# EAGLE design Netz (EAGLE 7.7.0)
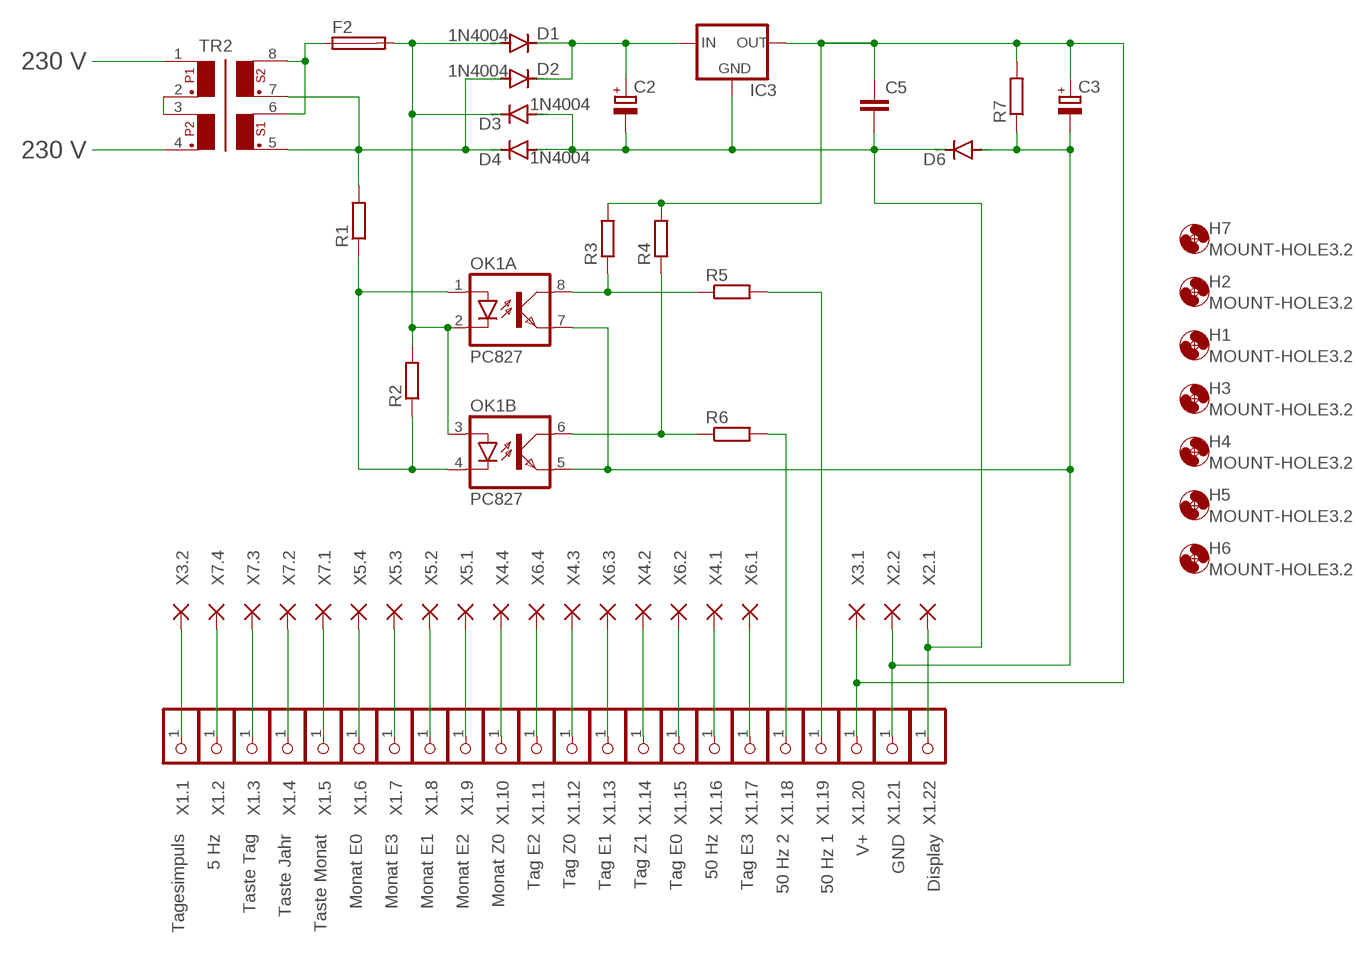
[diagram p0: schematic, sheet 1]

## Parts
C2  CPOL-EUE7.5-18  [E7,5-18]
C3  CPOL-EUE5-13  [E5-13]
C5  C-EU050-024X044  [C050-024X044]
D1  1N4004  [DO41-10]
D2  1N4004  [DO41-10]
D3  1N4004  [DO41-10]
D4  1N4004  [DO41-10]
D6  1N4148DO35-10  [DO35-10]
F2  SH22,5  [SH22,5]
H1  MOUNT-HOLE3.2  [3,2]
H2  MOUNT-HOLE3.2  [3,2]
H3  MOUNT-HOLE3.2  [3,2]
H4  MOUNT-HOLE3.2  [3,2]
H5  MOUNT-HOLE3.2  [3,2]
H6  MOUNT-HOLE3.2  [3,2]
H7  MOUNT-HOLE3.2  [3,2]
IC3  78XXS  [78XXS]
OK1  PC827  [DIL08]
R1  R-EU_0207/10  [0207/10]
R2  R-EU_0207/10  [0207/10]
R3  R-EU_0207/10  [0207/10]
R4  R-EU_0207/10  [0207/10]
R5  R-EU_0207/10  [0207/10]
R6  R-EU_0207/10  [0207/10]
R7  R-EU_0207/10  [0207/10]
TR2  FL02  [FL02-08]
X1.1  Tagesimpuls  PINHD-1X1  [1X01]
X1.2  5 Hz  PINHD-1X1  [1X01]
X1.3  Taste Tag  PINHD-1X1  [1X01]
X1.4  Taste Jahr  PINHD-1X1  [1X01]
X1.5  Taste Monat  PINHD-1X1  [1X01]
X1.6  Monat E0  PINHD-1X1  [1X01]
X1.7  Monat E3  PINHD-1X1  [1X01]
X1.8  Monat E1  PINHD-1X1  [1X01]
X1.9  Monat E2  PINHD-1X1  [1X01]
X1.10  Monat Z0  PINHD-1X1  [1X01]
X1.11  Tag E2  PINHD-1X1  [1X01]
X1.12  Tag Z0  PINHD-1X1  [1X01]
X1.13  Tag E1  PINHD-1X1  [1X01]
X1.14  Tag Z1  PINHD-1X1  [1X01]
X1.15  Tag E0  PINHD-1X1  [1X01]
X1.16  50 Hz  PINHD-1X1  [1X01]
X1.17  Tag E3  PINHD-1X1  [1X01]
X1.18  50 Hz 2  PINHD-1X1  [1X01]
X1.19  50 Hz 1  PINHD-1X1  [1X01]
X1.20  V+  PINHD-1X1  [1X01]
X1.21  GND  PINHD-1X1  [1X01]
X1.22  Display  PINHD-1X1  [1X01]
X2.1  WIREPAD1,6/0,8  [1,6/0,8]
X2.2  WIREPAD1,6/0,8  [1,6/0,8]
X3.1  WIREPAD1,6/0,8  [1,6/0,8]
X3.2  WIREPAD1,6/0,8  [1,6/0,8]
X4.1  WIREPAD1,6/0,8  [1,6/0,8]
X4.2  WIREPAD1,6/0,8  [1,6/0,8]
X4.3  WIREPAD1,6/0,8  [1,6/0,8]
X4.4  WIREPAD1,6/0,8  [1,6/0,8]
X5.1  WIREPAD1,6/0,8  [1,6/0,8]
X5.2  WIREPAD1,6/0,8  [1,6/0,8]
X5.3  WIREPAD1,6/0,8  [1,6/0,8]
X5.4  WIREPAD1,6/0,8  [1,6/0,8]
X6.1  WIREPAD1,6/0,8  [1,6/0,8]
X6.2  WIREPAD1,6/0,8  [1,6/0,8]
X6.3  WIREPAD1,6/0,8  [1,6/0,8]
X6.4  WIREPAD1,6/0,8  [1,6/0,8]
X7.1  WIREPAD1,6/0,8  [1,6/0,8]
X7.2  WIREPAD1,6/0,8  [1,6/0,8]
X7.3  WIREPAD1,6/0,8  [1,6/0,8]
X7.4  WIREPAD1,6/0,8  [1,6/0,8]

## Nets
N$1: D1.A D3.C F2.2 OK1.2(A:C) OK1.3(B:A) R2.2
N$2: F2.1 TR2.6 TR2.8
N$3: R5.2 X1.19.1
N$4: D2.A D4.C R1.2 TR2.5 TR2.7
N$5: C2.+ D1.C D2.C IC3.IN
N$6: R6.2 X1.18.1
N$7: X1.11.1 X6.4.1(P)
N$9: TR2.2 TR2.3
N$10: TR2.1
N$11: TR2.4
N$12: OK1.1(A:A) OK1.4(B:C) R1.1 R2.1
N$13: X1.13.1 X6.3.1(P)
N$14: OK1.8(A:COL) R3.1 R5.1
N$15: C2.- C5.2 D3.A D4.A D6.C IC3.GND X1.22.1 X2.1.1(P)
N$16: OK1.6(B:COL) R4.1 R6.1
N$17: C3.+ C5.1 IC3.OUT R3.2 R4.2 R7.2 X1.20.1 X3.1.1(P)
N$18: X1.15.1 X6.2.1(P)
N$19: X1.14.1 X4.2.1(P)
N$20: X1.12.1 X4.3.1(P)
N$21: X1.17.1 X6.1.1(P)
N$22: X1.16.1 X4.1.1(P)
N$23: X1.10.1 X4.4.1(P)
N$24: X1.6.1 X5.4.1(P)
N$25: X1.7.1 X5.3.1(P)
N$26: X1.8.1 X5.2.1(P)
N$27: X1.9.1 X5.1.1(P)
N$28: X1.4.1 X7.2.1(P)
N$29: X1.1.1 X3.2.1(P)
N$30: X1.5.1 X7.1.1(P)
N$31: X1.3.1 X7.3.1(P)
N$32: X1.2.1 X7.4.1(P)
N$33: C3.- D6.A OK1.5(B:EMIT) OK1.7(A:EMIT) R7.1 X1.21.1 X2.2.1(P)

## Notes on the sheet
- 230 V
- 230 V

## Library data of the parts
C2 C3 = rclxrund:CPOL-EU: POLARIZED CAPACITOR, European symbol; SPICEPREFIX: C
C5 = rclxrund:C-EU: CAPACITOR, European symbol; SPICEPREFIX: C
D1-D4 = diodexrund:1N4004: DIODE
D6 = diodexrund:1N4148: DIODE
F2 = fuserund:SH22,5: FUSE HOLDER; MF: SCHURTER; MPN: 0031.8201; OC_FARNELL: 1162740; OC_NEWARK: 96F8317
H1-H7 = holes:MOUNT-HOLE: MOUNTING HOLE with drill center marker
IC3 = v-regrund:78XXS: VOLTAGE REGULATOR
OK1 = optocouplerxrund:PC827: SHARP OPTO COUPLER; OC_FARNELL: unknown; OC_NEWARK: unknown
R1-R7 = rclxrund:R-EU_: RESISTOR, European symbol; SPICEPREFIX: R
TR2 = trafox:FL02: TRANSFORMER 2 primary winding, 2 secondary windings, mounting holes BLOCK
X1.1-X1.22 = pinheadxrund:PINHD-1X1: PIN HEADER
X2.1 X2.2 X3.1 X3.2 X4.1-X4.4 X5.1-X5.4 X6.1-X6.4 X7.1-X7.4 = wirepad:WIREPAD: Wire PAD connect wire on PCB

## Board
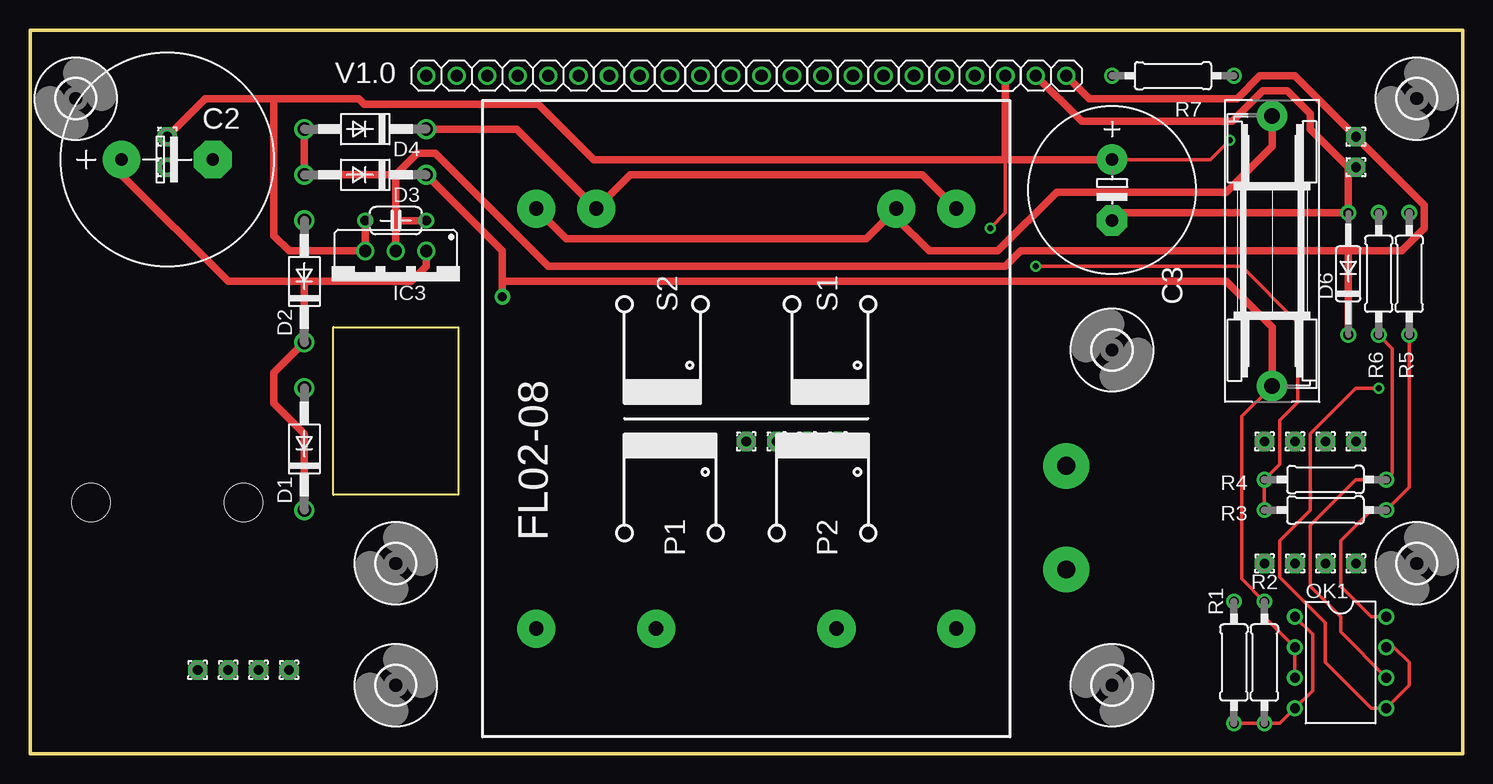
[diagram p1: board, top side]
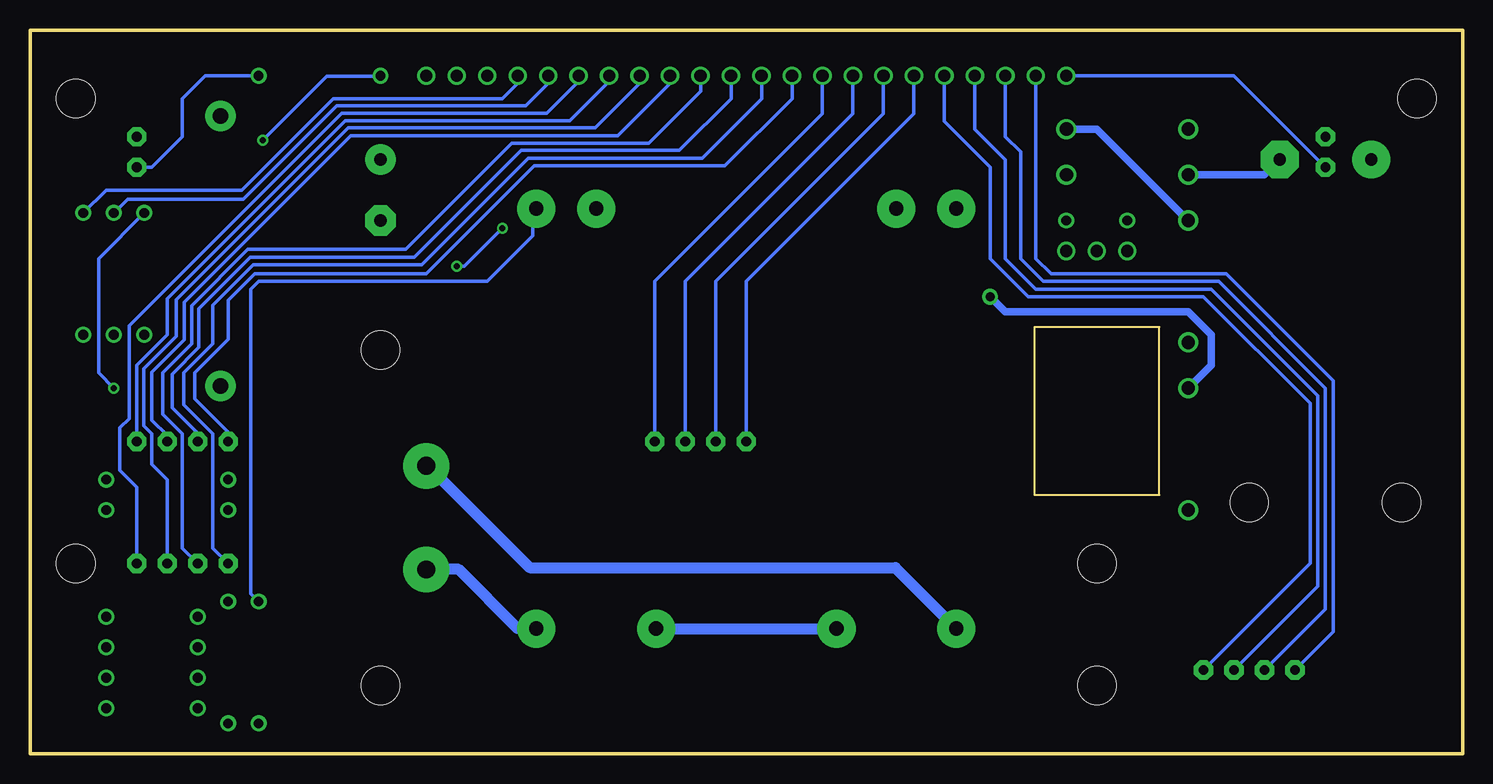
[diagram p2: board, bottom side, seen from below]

Size 119.38 x 60.33 mm. Coordinates in mm from the lower left corner, seen from the top.
Outline: 0,0 119.38,0 119.38,60.33 0,60.33 0,0
Copper layers (1*16): Top 0.035mm / dielectric 1.5mm / Bottom 0.035mm
Design rules "12mil": minimum track width 12mil, minimum drill 0.5mm, track to track 12mil, track to pad 12mil, pad to pad 12mil, via to via 12mil, smd to smd 6mil, copper to edge 40mil, drill to drill 12mil, minimum pad ring 10mil, minimum via ring 8mil, stop-mask expansion 4mil, vias tented up to drill 0mil, thermal gap 10mil
Holes 3.17 mm at 5.08,20.95 17.78,20.95
Milling: 4 lines

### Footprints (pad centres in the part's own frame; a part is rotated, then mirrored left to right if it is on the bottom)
E7,5-18 = drill 1.016 pad 3.15: + -3.81,0 | drill 1.016 pad 3.15 octagon: - 3.81,0
E5-13 = drill 1.016 pad 2.54: + -2.54,0 | drill 1.016 pad 2.54 octagon: - 2.54,0
C050-024X044 = drill 0.813: 1 -2.54,0; 2 2.54,0
DO41-10 = drill 1.118: A 5.08,0; C -5.08,0
DO35-10 = drill 0.813: A 5.08,0; C -5.08,0
SH22,5 = drill 1.321 pad 2.54: 1 -11.252,0; 2 11.252,0
3,2 = hole 3.2: 0,0
78XXS = drill 1.016: GND 0,-2.54; IN -2.54,-2.54; OUT 2.54,-2.54
DIL08 = drill 0.813: 1 -3.81,-3.81; 2 -1.27,-3.81; 3 1.27,-3.81; 4 3.81,-3.81; 5 3.81,3.81; 6 1.27,3.81; 7 -1.27,3.81; 8 -3.81,3.81
0207/10 = drill 0.813: 1 -5.08,0; 2 5.08,0
FL02-08 = drill 1.194 pad 3.175: 1 -17.501,17.501; 2 -17.501,7.518; 3 -17.501,-7.518; 4 -17.501,-17.501; 5 17.501,-17.501; 6 17.501,-12.497; 7 17.501,12.497; 8 17.501,17.501
1X01 = drill 1.016: 1 0,0
1,6/0,8 = drill 0.813 pad 1.6 octagon: 1 0,0

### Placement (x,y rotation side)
C2  11.43,49.53 0 top
C3  90.17,46.99 270 top
C5  30.48,44.45 0 top
D1  22.86,25.4 90 top
D2  22.86,39.37 90 top
D3  27.94,48.26 180 top
D4  27.94,52.07 180 top
D6  109.86,40.01 90 top
F2  103.5,41.91 270 top
H1  30.48,15.88 0 top
H2  30.48,5.71 0 top
H3  3.81,54.61 0 top
H4  115.57,54.61 0 top
H5  90.17,5.71 90 top
H6  90.17,33.66 90 top
H7  115.57,15.88 0 top
IC3  30.48,39.37 180 top
OK1  109.22,7.62 270 top
R1  100.33,7.62 90 top
R2  102.87,7.62 90 top
R3  107.95,20.32 180 top
R4  107.95,22.86 180 top
R5  114.94,40.01 90 top
R6  112.39,40.01 90 top
R7  95.25,56.52 180 top
TR2  59.69,27.94 90 top
X1.1  33.02,56.52 0 top
X1.2  35.56,56.52 0 top
X1.3  38.1,56.52 0 top
X1.4  40.64,56.52 0 top
X1.5  43.18,56.52 0 top
X1.6  45.72,56.52 0 top
X1.7  48.26,56.52 90 top
X1.8  50.8,56.52 90 top
X1.9  53.34,56.52 90 top
X1.10  55.88,56.52 90 top
X1.11  58.42,56.52 90 top
X1.12  60.96,56.52 90 top
X1.13  63.5,56.52 90 top
X1.14  66.04,56.52 90 top
X1.15  68.58,56.52 90 top
X1.16  71.12,56.52 90 top
X1.17  73.66,56.52 90 top
X1.18  76.2,56.52 180 top
X1.19  78.74,56.52 180 top
X1.20  81.28,56.52 90 top
X1.21  83.82,56.52 180 top
X1.22  86.36,56.52 90 top
X2.1  110.49,51.44 0 top
X2.2  110.49,48.9 0 top
X3.1  11.43,51.44 0 top
X3.2  11.43,48.9 0 top
X4.1  110.49,26.04 0 top
X4.2  107.95,26.04 0 top
X4.3  105.41,26.04 0 top
X4.4  102.87,26.04 0 top
X5.1  67.31,26.04 0 top
X5.2  64.77,26.04 0 top
X5.3  62.23,26.04 0 top
X5.4  59.69,26.04 0 top
X6.1  110.49,15.88 0 top
X6.2  107.95,15.88 0 top
X6.3  105.41,15.88 0 top
X6.4  102.87,15.88 0 top
X7.1  21.59,6.99 0 top
X7.2  19.05,6.99 0 top
X7.3  16.51,6.99 0 top
X7.4  13.97,6.99 0 top

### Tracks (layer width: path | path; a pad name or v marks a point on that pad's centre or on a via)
N$1  (via drill 0.75 pad 1.3)
  Top 0.305: F2.2 100.97,28.12 100.97,14.61 R2.2 102.87,11.43 OK1.2 OK1.3
  Top 0.61: D3.C 39.37,41.91 39.37,39.37 | v39.37,38.1 39.37,39.37 | F2.2 103.5,35.56 99.69,39.37 39.37,39.37
  Bottom 0.61: v39.37,38.1 38.1,36.83 22.86,36.83 20.95,34.92 20.95,32.38 D1.A
N$2
  Top 0.61: TR2.8 44.69,42.94 69.69,42.94 TR2.6 72.19,44.65 74.93,41.91 80.64,41.91 85.55,46.81 99.69,46.81 103.5,50.62 F2.1
N$3
  Bottom 0.305: X1.19.1 78.74,55.88 80.01,54.61 94.11,54.61 101.73,46.99 113.03,46.99 R5.2
N$4
  Top 0.61: TR2.5 74.37,48.26 50.01,48.26 TR2.7 40.56,52.07 D4.C
  Bottom 0.305: R1.2 100.97,13.34 100.97,38.73 100.33,39.37 81.28,39.37 77.47,43.18 77.47,45.16 TR2.5
  Bottom 0.61: D2.A 30.48,52.07 D4.C
N$5
  Top 0.61: IC3.IN 33.02,40.64 31.75,39.37 22.86,39.37 | 22.86,39.37 D2.C 20.32,31.75 20.32,29.21 22.86,26.67 D1.C | 22.86,39.37 16.51,39.37 7.62,48.26 C2.+
N$6
  Bottom 0.305: R6.2 112.37,45.09 111.23,46.23 101.6,46.23 93.83,54 78.08,54 76.2,55.88 X1.18.1
N$7
  Bottom 0.305: X6.4.1 104.14,17.14 104.14,26.7 106.55,29.11 106.55,31.75 104.14,34.16 104.14,37.39 100.77,40.77 86.74,40.77 77.85,49.66 63.37,49.66 58.42,54.61 X1.11.1
N$9
  Bottom 0.914: TR2.3 TR2.2
N$10  (via drill 1.5 pad 3.81)
  Bottom 0.914: TR2.1 47.27,15.52 77.75,15.52 86.23,24 v86.36,24
N$11  (via drill 1.5 pad 3.81)
  Bottom 0.914: TR2.4 78.74,10.44 83.67,15.37 v86.36,15.37
N$12
  Top 0.305: OK1.1 106.88,9.96 106.88,5.28 OK1.4 104.14,2.54 R2.1 R1.1
N$13
  Bottom 0.305: X1.13.1 63.5,55.22 67.82,50.9 79.22,50.9 88.08,42.04 101.22,42.04 105.92,37.34 105.92,34.16 108.33,31.75 108.33,28.32 106.68,26.67 106.68,17.14 X6.3.1
N$14
  Top 0.305: R5.1 114.94,22.23 R3.1 111.76,20.32 109.22,17.78 109.22,13.97 111.76,11.43 OK1.8
N$15
  Top 0.61: IC3.GND 30.48,44.45 | D4.A D3.A 30.48,48.26 | 30.48,44.45 C5.2 | 30.48,44.45 30.48,48.26 | 109.86,41.91 D6.C | 109.86,41.91 82.55,41.91 81.28,40.64 43.18,40.64 33.78,50.04 32.26,50.04 30.48,48.26 | 109.86,41.91 114.3,41.91 116.2,43.81 116.2,45.72 X2.1.1 105.41,56.52 102.49,56.52 100.58,54.61 88.27,54.61 X1.22.1
  Bottom 0.61: D3.A 16.51,48.26 C2.-
N$16
  Top 0.305: R6.1 113.54,33.78 113.54,23.37 R4.1 110.49,22.86 106.68,19.05 106.68,13.97 109.22,11.43 109.22,10.16 OK1.6
N$17  (via drill 0.5)
  Top 0.305: R3.2 R4.2 104.14,24.13 104.14,27.78 105.66,29.31 105.66,35.94 100.97,40.64 v83.82,40.64 | 81.28,49.53 81.28,45.09 v80.01,43.81 | v99.98,51.15 98.37,49.53 C3.+
  Top 0.61: C5.1 IC3.OUT 21.59,41.91 20.32,43.18 20.32,54.61 | C3.+ 81.28,49.53 | 81.28,49.53 46.99,49.53 42.37,54.15 27.86,54.15 27.4,54.61 20.32,54.61 | X1.20.1 81.28,49.53 | 20.32,54.61 14.61,54.61 X3.1.1
  Bottom 0.305: v83.82,40.64 83.19,40.64 v80.01,43.81 | v99.98,51.15 94.65,56.48 90.21,56.48 R7.2
N$18
  Bottom 0.305: X1.15.1 68.58,55.88 72.29,52.17 92.86,52.17 107.19,37.85 107.19,34.8 109.88,32.11 109.88,27.33 109.22,26.67 109.22,24.13 107.95,22.86 X6.2.1
N$19
  Bottom 0.305: X1.14.1 66.04,55.88 70.41,51.51 92.66,51.51 106.53,37.65 106.53,34.52 109.22,31.82 109.22,27.81 107.95,26.54 X4.2.1
N$20
  Bottom 0.305: X4.3.1 105.41,26.72 107.54,28.86 107.54,31.65 105.31,33.88 105.31,37.09 101.02,41.38 87.38,41.38 78.46,50.29 65.28,50.29 60.96,54.61 X1.12.1
N$21
  Bottom 0.305: X6.1.1 110.49,22.23 111.89,23.62 111.89,27.18 111.12,27.94 111.12,35.69 93.42,53.39 76.33,53.39 73.66,56.06 X1.17.1
N$22
  Bottom 0.305: X4.1.1 110.49,32.38 107.95,34.92 107.95,37.95 93.12,52.78 74.4,52.78 71.12,56.06 X1.16.1
N$23
  Bottom 0.305: X4.4.1 102.87,26.8 105.66,29.59 105.66,31.75 102.87,34.54 102.87,37.8 100.67,40.01 86.36,40.01 77.34,49.02 61.47,49.02 55.88,54.61 X1.10.1
N$24
  Bottom 0.305: X1.6.1 45.72,53.34 59.69,39.37 X5.4.1
N$25
  Bottom 0.305: X1.7.1 48.26,53.34 62.23,39.37 X5.3.1
N$26
  Bottom 0.305: X1.8.1 50.8,53.34 64.77,39.37 X5.2.1
N$27
  Bottom 0.305: X1.9.1 53.34,53.34 67.31,39.37 X5.1.1
N$28
  Bottom 0.305: X1.4.1 40.64,52.07 38.1,49.53 38.1,41.27 35.56,38.73 20.95,38.73 12.06,29.84 12.06,13.97 X7.2.1
N$29
  Bottom 0.305: X3.2.1 19.05,56.52 X1.1.1
N$30
  Bottom 0.305: X1.5.1 43.18,52.7 39.37,48.9 39.37,41.27 36.2,38.1 21.59,38.1 12.7,29.21 12.7,15.88 X7.1.1
N$31
  Bottom 0.305: X1.3.1 38.1,51.44 36.83,50.16 36.83,41.27 34.92,39.37 20.32,39.37 11.43,30.48 11.43,12.06 X7.3.1
N$32
  Bottom 0.305: X7.4.1 10.79,10.16 10.79,31.11 19.68,40.01 34.29,40.01 35.56,41.27 X1.2.1
N$33  (via drill 0.5)
  Top 0.305: OK1.7 113.67,8.89 114.94,7.62 114.94,5.71 OK1.5 111.76,3.81 107.95,7.62 107.95,10.92 104.14,14.73 104.14,17.78 106.68,20.32 106.68,26.67 110.49,30.48 v112.39,30.48
  Top 0.61: C3.- 90.81,45.09 D6.A 109.86,48.9 | 109.86,48.9 X2.2.1 | 109.86,48.9 106.68,52.07 106.68,53.34 104.78,55.24 102.74,55.24 100.2,52.7 87.63,52.7 X1.21.1
  Bottom 0.305: D6.A 113.67,41.27 113.67,31.75 v112.39,30.48 | R7.1 104.78,56.52 106.68,54.61 106.68,51.44 109.22,48.9 X2.2.1

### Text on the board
tPlace: V1.0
